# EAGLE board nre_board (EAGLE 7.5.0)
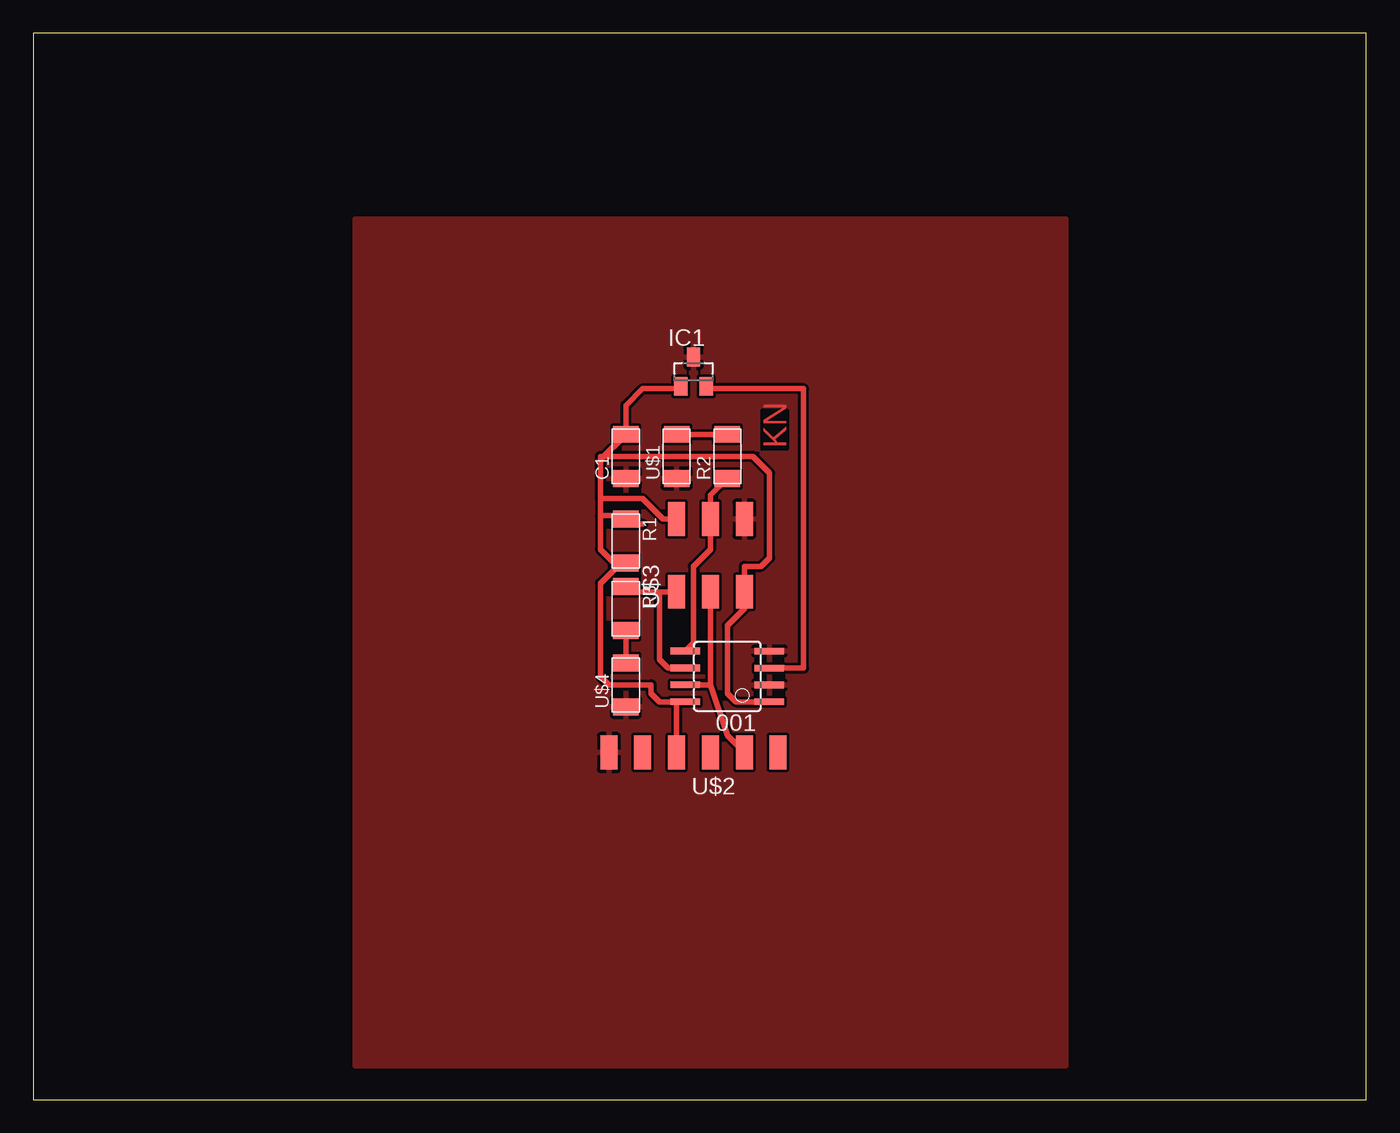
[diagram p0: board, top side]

Size 100 x 80 mm. Coordinates in mm from the lower left corner, seen from the top.
Outline: 0,0 100,0 100,80 0,80 0,0
Copper layers (1*16): Top 0.035mm / dielectric 1.5mm / Bottom 0.035mm
Design rules "default": minimum track width 10mil, minimum drill 24mil, track to track 8mil, track to pad 8mil, pad to pad 8mil, via to via 8mil, smd to smd 8mil, copper to edge 40mil, drill to drill 8mil, minimum pad ring 10mil, minimum via ring 8mil, stop-mask expansion 4mil, vias tented up to drill 0mil, thermal gap 10mil

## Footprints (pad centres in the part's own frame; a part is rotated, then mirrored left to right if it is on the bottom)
SOIC8 = smd 0.5 x 2.2: 1 -1.905,-3.154; 2 -0.645,-3.154; 3 0.625,-3.154; 4 1.895,-3.154; 5 1.905,3.154; 6 0.635,3.154; 7 -0.635,3.154; 8 -1.905,3.154
C1206FAB = smd 1.27 x 1.905: 1 -1.651,0; 2 1.651,0
SOT23 = smd 1 x 1.4: 1 -0.95,-1.1; 2 0.95,-1.1; 3 0,1.1
R1206FAB = smd 1.27 x 1.905: 1 -1.651,0; 2 1.651,0
LED1206FAB = smd 1.27 x 1.905: 1 -1.651,0; 2 1.651,0
1X06SMD = smd 2.54 x 1.27: 1 0,6.35; 2 0,3.81; 3 0,1.27; 4 0,-1.27; 5 0,-3.81; 6 0,-6.35
2X03SMD = smd 2.54 x 1.27: 1 -2.54,2.54; 2 2.92,2.54; 3 -2.54,0; 4 2.92,0; 5 -2.54,-2.54; 6 2.92,-2.54

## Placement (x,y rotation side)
001  ATTINY45SI  [SOIC8]  52.07,31.75 90 top
C1  CAP-US1206FAB  [C1206FAB]  44.45,48.26 90 top
IC1  A1324-HALL-SENSOR  [SOT23]  49.53,54.61 0 top
R1  [R1206FAB]  44.45,41.91 270 top
R2  499  [R1206FAB]  52.07,48.26 90 top
R3  499  [R1206FAB]  44.45,36.83 270 top
U$1  LEDFAB1206  [LED1206FAB]  48.26,48.26 90 top
U$2  FTDI-SMD-HEADER  [1X06SMD]  49.53,26.04 90 top
U$3  AVRISPSMD  [2X03SMD]  50.8,40.64 90 top
U$4  LEDFAB1206  [LED1206FAB]  44.45,31.11 90 top

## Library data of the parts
001 C1 IC1 R1 U$2 U$3 = fab
R2 R3 U$1 U$4 = fablab

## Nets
GND: 001.2 001.4 C1.1 IC1.3 U$1.1 U$2.1 U$3.6 U$4.1
MISO: 001.6 R3.1 U$3.1
MOSI: 001.5 R2.1 U$3.4
N$1: 001.7 U$2.5 U$3.3
N$2: 001.1 R1.1 U$3.5
N$4: 001.3 IC1.2
N$6: R2.2 U$1.2
N$8: R3.2 U$4.2
VCC: 001.8 C1.2 IC1.1 R1.2 U$2.3 U$3.2

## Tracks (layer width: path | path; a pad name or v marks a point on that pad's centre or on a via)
GND
  pour Top: 24.13,66.04 77.47,66.04 77.47,2.54 24.13,2.54 24.13,3.81
MISO
  Top 0.406: U$3.1 46.99,38.1 | 46.99,38.1 44.83,38.1 R3.1 | 001.6 47.62,32.38 46.99,33.02 46.99,38.1
MOSI
  Top 0.406: R2.1 50.8,45.34 U$3.4 50.8,41.27 49.53,40.01 49.53,34.27 001.5
N$1
  Top 0.406: 001.7 50.8,31.11 | 50.8,31.11 52.07,27.3 U$2.5 | U$3.3 50.8,31.11
N$2
  Top 0.406: 45.72,43.18 44.83,43.18 R1.1 44.2,43.81 42.55,43.81 42.55,48.26 53.98,48.26 55.24,46.99 55.24,40.64 54.61,40.01 53.34,40.01 U$3.5 53.34,36.83 52.07,35.56 52.07,30.48 52.7,29.84 53.98,29.84 54.61,29.84 001.1
N$4
  Top 0.406: 001.3 57.78,32.38 57.78,53.34 50.48,53.34 IC1.2
N$6
  Top 0.406: U$1.2 R2.2
N$8
  Top 0.406: U$4.2 R3.2
VCC
  Top 0.406: 001.8 48.26,29.84 | 48.26,29.84 U$2.3 | U$3.2 47.24,43.56 45.72,45.09 42.55,45.09 | 42.55,45.09 42.55,41.27 43.81,40.01 | R1.2 44.2,40.01 43.81,40.01 | 43.81,40.01 42.55,38.73 42.55,31.75 43.18,31.11 46.35,31.11 46.35,30.48 46.99,29.84 48.26,29.84 | 42.55,45.09 42.55,48.01 C1.2 44.45,52.07 45.72,53.34 48.41,53.34 IC1.1

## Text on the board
Top: KN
